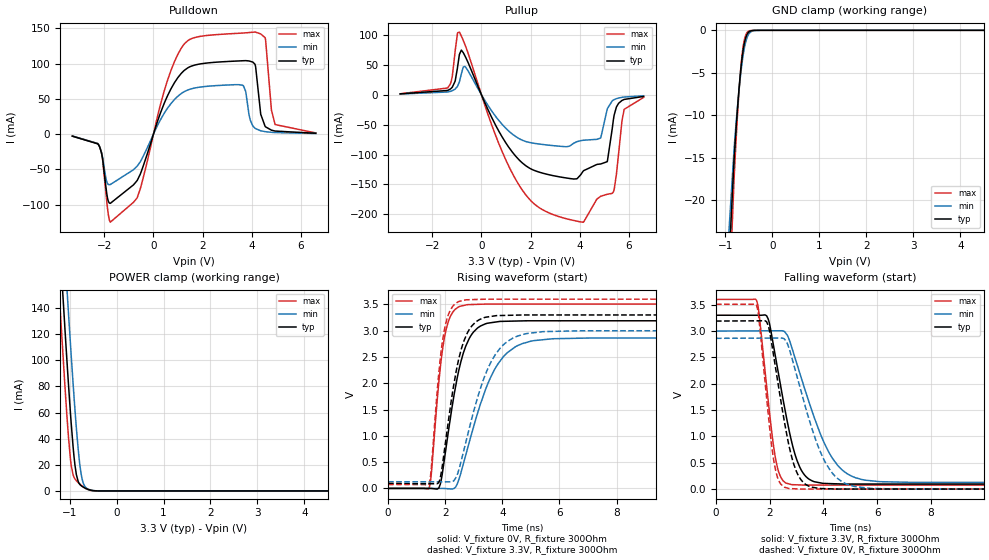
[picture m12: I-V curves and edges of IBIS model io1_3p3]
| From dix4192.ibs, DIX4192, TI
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|   io1_3p3 Model
[Model]   io1_3p3
Model_type   I/O
Polarity   Non-Inverting
Enable   Active-Low
Vinl = 0.99
Vinh = 2.31
Vmeas = 1.65
Vref = 0
Cref = 2pF
Rref = 100000
|   typ   min   max
C_comp   31.0199pF   25.2142pF   36.9522pF
|C_comp_pullup   31.4512pF   25.5647pF   37.4639pF
|C_comp_pulldown   31.7418pF   25.9171pF   37.6378pF
[Model spec]
|subparameter
Vinl   0.99   0.90   1.08
Vinh   2.31   2.10   2.52
| Where nom  PVT is Nominal Process, 3.3V, 27C
|   Fast PVT is Strong Process,  3.6V, -40C
|   Slow PVT is Weak Process,   3.0V, 105C
[Voltage Range]   3.3   3   3.6
[Temperature Range]   27   105   -40
[Pullup Reference]   3.3   3   3.6
[Pulldown Reference]   -0   0   0
[Power Clamp Reference]   3.3   3   3.6
[GND Clamp Reference]   0   0   0
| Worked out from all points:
|   slope of the pulldown table from 0 to 0.495 V, typ, clamps not added: 10.2 ohm
|   slope of the pullup table from 0 to 0.495 V, typ, clamps not added: 11.2 ohm
|   GND clamp passes 1 mA (typ) near -0.57 V on its own axis
|   POWER clamp passes 1 mA (typ) near -0.59 V on its own axis
|   falling waveform, V_fixture 3.3V, R_fixture 300Ohm: 20-80 % time 736ps typ, 1.22ns min, 460ps max; typ from 3.3 V to 0.095 V
|   rising waveform, V_fixture 0V, R_fixture 300Ohm: 20-80 % time 628ps typ, 1.07ns min, 377ps max; typ from 0 V to 3.19 V
|   rising waveform, V_fixture 3.3V, R_fixture 300Ohm: 20-80 % time 593ps typ, 985ps min, 362ps max; typ from 0.095 V to 3.3 V
|   falling waveform, V_fixture 0V, R_fixture 300Ohm: 20-80 % time 666ps typ, 1.07ns min, 425ps max; typ from 3.19 V to 0 V
[Pulldown]
|   Voltage   I(typ)   I(min)   I(max)
-3.3V     -2.852mA   -2.596mA   -2.853mA
-2.191V   -18.1mA    -17.63mA   -17.6mA
-1.756V   -98.08mA   -71.43mA   -124.8mA
-656.7mV  -65.33mA   -45.07mA   -89.62mA
432.3mV   43.23mA    29.27mA    60.55mA
1.214V    89.07mA    59.43mA    126mA
3.64V     104mA      68.94mA    143.3mA
4.125V    99.15mA    8.551mA    144.6mA
4.551V    10.64mA    3.483mA    135.2mA
4.798V    5.618mA    2.568mA    34.1mA
4.947V    4.357mA    2.216mA    13.59mA
6.6V      1.224mA    869.1uA    1.663mA
[GND Clamp]
|   Voltage   I(typ)   I(min)   I(max)
-3.3V     -1.043A    -967.2mA   -1.114A
-1.152V   -52.44mA   -43.82mA   -63.48mA
-815.1mV  -15.28mA   -13.99mA   -17.55mA
-765.6mV  -11.04mA   -10.51mA   -12.26mA
-726mV    -8.028mA   -7.997mA   -8.54mA
-686.4mV  -5.443mA   -5.78mA    -5.412mA
-656.7mV  -3.831mA   -4.343mA   -3.536mA
-627mV    -2.532mA   -3.123mA   -2.114mA
-587.4mV  -1.301mA   -1.859mA   -911.7uA
-498.3mV  -181.2uA   -403.3uA   -76.67uA
-260.7mV  0A         -988.6nA   0A
6.6V      0A         0A         0A
[Pullup]
|   Voltage   I(typ)   I(min)   I(max)
-3.3V     1.193mA    955.2uA    1.362mA
-1.369V   6.903mA    4.325mA    11mA
-1.073V   21.93mA    9.068mA    70.24mA
-894.3mV  66.92mA    21.2mA     104.3mA
-646.8mV  62.78mA    45.89mA    81.1mA
1.601V    -111.6mA   -74.87mA   -155.5mA
4.135V    -128mA     -76.26mA   -212.9mA
4.848V    -115.8mA   -72.43mA   -169.8mA
5.115V    -112mA     -24.76mA   -166.3mA
5.362V    -43.87mA   -9.266mA   -162.9mA
5.808V    -8.057mA   -4.053mA   -24.56mA
6.6V      -3.083mA   -1.984mA   -4.668mA
[POWER Clamp]
|   Voltage   I(typ)   I(min)   I(max)
-3.3V     1.547A     1.6A       1.506A
-1.261V   221.8mA    278.9mA    176.5mA
-1.201V   185.4mA    242.4mA    140.3mA
-1.181V   173.4mA    230.3mA    128.4mA
-1.092V   120.7mA    176.8mA    76.94mA
-1.063V   103.7mA    159.3mA    60.97mA
-1.033V   87.14mA    142.1mA    46.08mA
-963.6mV  51.24mA    103.1mA    19.41mA
-854.7mV  12.41mA    48.08mA    7.805mA
-745.8mV  3.823mA    11.52mA    4.15mA
-607.2mV  1.171mA    1.445mA    1.051mA
6.6V      0A         0A         0A
[Ramp]
R_load = 300
|   typ   min   max
dV/dt_r   1.91352/6.27551e-10   1.71722/1.06984e-09   2.10458/3.75844e-10
dV/dt_f   1.92296/7.34247e-10   1.72388/1.21792e-09   2.11532/4.59511e-10
[Falling Waveform]
V_fixture = 3.3V
V_fixture_min = 3V
V_fixture_max = 3.6V
R_fixture = 300Ohm
C_fixture = 0F
|   Time   V(typ)   V(min)   V(max)
0s        3.3V       3V         3.6V
1.512ns   3.3V       3.003V     3.579V
1.939ns   3.235V     3.004V     1.704V
2.232ns   2.465V     3.005V     541.8mV
2.446ns   1.853V     3.006V     197.9mV
2.815ns   904.5mV    2.7V       85.97mV
3.347ns   241.1mV    1.837V     76.74mV
4.228ns   105.8mV    678mV      76.74mV
5.549ns   97.48mV    171.4mV    76.74mV
50ns      95.07mV    126.9mV    74.47mV
[Rising Waveform]
V_fixture = 0V
V_fixture_min = 0V
V_fixture_max = 0V
R_fixture = 300Ohm
C_fixture = 0F
|   Time   V(typ)   V(min)   V(max)
0s        -1.246uV   -601.7nV   -859.3nV
1.427ns   291.4uV    128.7uV    -3.283mV
1.775ns   5.364mV    160.2uV    2.01V
1.98ns    583.4mV    -2.194mV   2.887V
2.366ns   1.942V     27.51mV    3.412V
2.77ns    2.765V     734.9mV    3.494V
3.464ns   3.138V     1.954V     3.505V
4.041ns   3.177V     2.507V     3.505V
5.772ns   3.187V     2.846V     3.505V
50ns      3.189V     2.862V     3.508V
[Rising Waveform]
V_fixture = 3.3V
V_fixture_min = 3V
V_fixture_max = 3.6V
R_fixture = 300Ohm
C_fixture = 0F
|   Time   V(typ)   V(min)   V(max)
0s        95.07mV    126.9mV    74.47mV
1.427ns   89.34mV    125.4mV    78.09mV
1.507ns   89.02mV    125.3mV    345.7mV
1.797ns   142.4mV    125mV      2.307V
1.964ns   691.1mV    124.9mV    2.999V
2.391ns   2.247V     217.7mV    3.526V
2.727ns   2.895V     888.6mV    3.586V
3.75ns    3.282V     2.541V     3.597V
5.426ns   3.298V     2.981V     3.597V
50ns      3.3V       3V         3.6V
[Falling Waveform]
|Gnd
V_fixture = 0V
V_fixture_min = 0V
V_fixture_max = 0V
R_fixture = 300Ohm
C_fixture = 0F
|   Time   V(typ)   V(min)   V(max)
0s        3.189V     2.862V     3.508V
1.512ns   3.194V     2.865V     3.485V
1.884ns   3.177V     2.866V     1.737V
2.174ns   2.446V     2.866V     477.5mV
2.384ns   1.777V     2.867V     118.1mV
2.727ns   808.9mV    2.666V     11.33mV
3.237ns   135.1mV    1.732V     2.296mV
4.108ns   8.635mV    474mV      2.294mV
5.772ns   2.349mV    13.79mV    2.29mV
50ns      -1.242uV   -600.5nV   -402.2nV
